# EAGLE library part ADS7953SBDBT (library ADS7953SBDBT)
12-Bit, 1-MSPS, 16-Channel, Single-Ended, microPower SAR ADC with Serial I/F Source: Datasheet
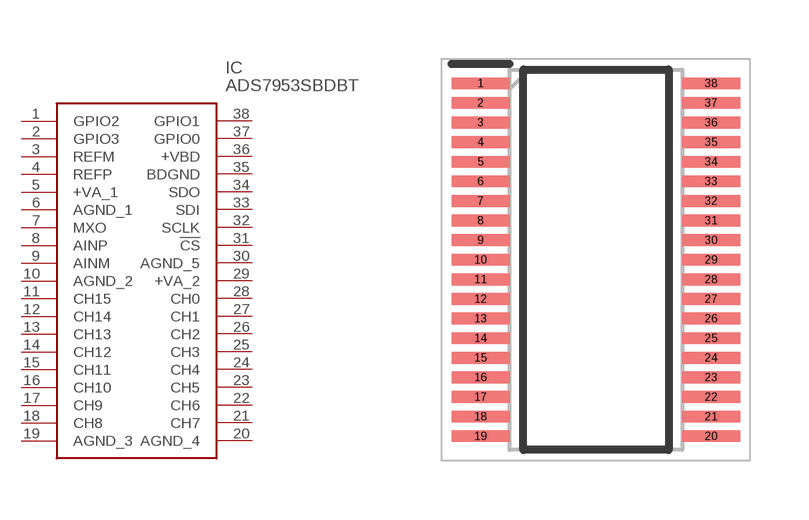
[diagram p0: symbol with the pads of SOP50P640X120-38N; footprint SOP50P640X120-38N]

Designator prefix IC

## ADS7953SBDBT (Description: 12-Bit, 1-MSPS, 16-Channel, Single-Ended, microPower SAR ADC with Serial I/F; Height: 1.2mm; Manufacturer_Name: Texas Instruments; Manufacturer_Part_Number: ADS7953SBDBT; Mouser_Part_Number: 595-ADS7953SBDBT; Mouser_Price-Stock: https://www.mouser.co.uk/ProductDetail/Texas-Instruments/ADS7953SBDBT?qs=Lv5%252BaqTFJEPgQ17SA2TUyg%3D%3D)  [SOP50P640X120-38N]
1  GPIO2
2  GPIO3
3  REFM
4  REFP
5  +VA_1
6  AGND_1
7  MXO
8  AINP
9  AINM
10  AGND_2
11  CH15
12  CH14
13  CH13
14  CH12
15  CH11
16  CH10
17  CH9
18  CH8
19  AGND_3
20  AGND_4
21  CH7
22  CH6
23  CH5
24  CH4
25  CH3
26  CH2
27  CH1
28  CH0
29  +VA_2
30  AGND_5
31  !CS
32  SCLK
33  SDI
34  SDO
35  BDGND
36  +VBD
37  GPIO0
38  GPIO1

## Footprint SOP50P640X120-38N (pad centres in mm)
DBT0038A
smd 1.475 x 0.3: 1 -2.938,4.5; 2 -2.938,4; 3 -2.938,3.5; 4 -2.938,3; 5 -2.938,2.5; 6 -2.938,2; 7 -2.938,1.5; 8 -2.938,1; 9 -2.938,0.5; 10 -2.938,0; 11 -2.938,-0.5; 12 -2.938,-1; 13 -2.938,-1.5; 14 -2.938,-2; 15 -2.938,-2.5; 16 -2.938,-3; 17 -2.938,-3.5; 18 -2.938,-4; 19 -2.938,-4.5; 20 2.938,-4.5; 21 2.938,-4; 22 2.938,-3.5; 23 2.938,-3; 24 2.938,-2.5; 25 2.938,-2; 26 2.938,-1.5; 27 2.938,-1; 28 2.938,-0.5; 29 2.938,0; 30 2.938,0.5; 31 2.938,1; 32 2.938,1.5; 33 2.938,2; 34 2.938,2.5; 35 2.938,3; 36 2.938,3.5; 37 2.938,4; 38 2.938,4.5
